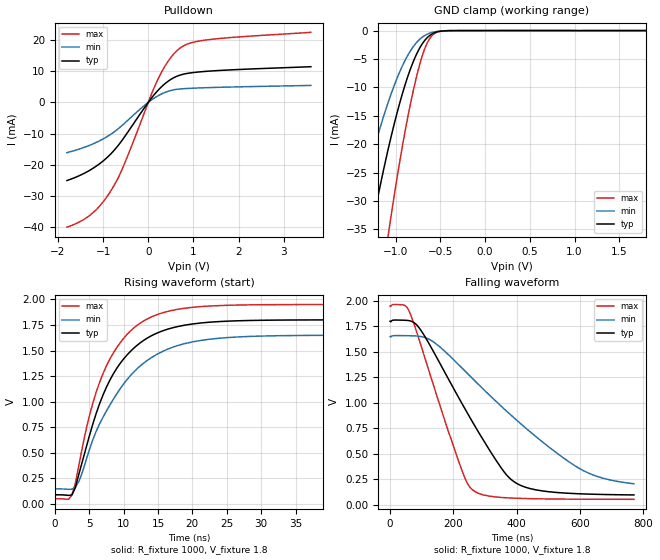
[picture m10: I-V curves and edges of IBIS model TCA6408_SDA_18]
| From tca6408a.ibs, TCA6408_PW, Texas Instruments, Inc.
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[Model]   TCA6408_SDA_18
Model_type  I/O_open_drain
Vinl=0.495
Vinh=1.365
Enable   Active-Low
Vref =   1.8
Rref =   1000
Cref =   50p
Vmeas =   0.9
| variable   typ   min   max
C_comp   2.96pF   1.98pF   3.47pF
| C_pulldown   1.93pF   0.86pF   2.70pF
| C_tri-state   2.96pF   1.98pF   3.47pF
[Temperature Range]   40   100   -40
| Ambient temperature   25   85   -40
[Voltage range]   1.8   1.65   1.95
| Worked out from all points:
|   slope of the pulldown table from 0 to 0.27 V, typ, clamps not added: 57.8 ohm
|   GND clamp passes 1 mA (typ) near -0.63 V on its own axis
|   rising waveform, R_fixture 1000, V_fixture 1.8: 20-80 % time 6.45ns typ, 7.78ns min, 5.79ns max; typ from 0.089 V to 1.8 V
|   falling waveform, R_fixture 1000, V_fixture 1.8: 20-80 % time 190ns typ, 311ns min, 119ns max; typ from 1.8 V to 0.094 V
[GND Clamp]
| TCA6408_SDA_18
|   Voltage   I(typ)   I(min)   I(max)
-1.8V     -85.23mA   -59.03mA   -129.6mA
-1.475V   -52.85mA   -35.21mA   -83.87mA
-1.275V   -35.29mA   -22.64mA   -58.08mA
-1.075V   -20.23mA   -12.2mA    -35.04mA
-965mV    -13.31mA   -7.618mA   -23.97mA
-860mV    -7.844mA   -4.209mA   -14.81mA
-760mV    -3.915mA   -1.979mA   -7.656mA
-675mV    -1.722mA   -861.6uA   -3.173mA
-630mV    -990.4uA   -511.7uA   -1.658mA
-585mV    -515uA     -286.9uA   -750uA
-455mV    -48.62uA   -37.39uA   -47.18uA
1.8V      212.6pA    1.031uA    -1.64uA
[Pulldown]
| TCA6408_SDA_18
|   Voltage   I(typ)   I(min)   I(max)
-1.8V     -25.03mA   -16.11mA   -39.97mA
-1.255V   -21.4mA    -13.49mA   -35.72mA
-1.045V   -19.29mA   -12.06mA   -32.67mA
-825mV    -16.44mA   -10.17mA   -28.24mA
-550mV    -11.55mA   -7.013mA   -20.47mA
60mV      1.174mA    652.4uA    2.253mA
215mV     3.846mA    2.097mA    7.413mA
445mV     6.827mA    3.573mA    13.29mA
680mV     8.622mA    4.255mA    17.11mA
920mV     9.403mA    4.495mA    18.95mA
1.315V    9.977mA    4.717mA    20.05mA
3.6V      11.43mA    5.425mA    22.44mA
[Ramp]
| TCA6408_SDA_18
| variable   typ   min   max
dV/dt_r   1.03/6.45E-09   0.90/7.78E-09   1.14/5.79E-09
dV/dt_f   1.03/1.91E-07   0.87/3.13E-07   1.15/1.20E-07
R_load = 1000
[Rising Waveform]
| TCA6408_SDA_18
R_fixture =   1000
C_fixture =   0
L_fixture =   0
V_fixture =   1.8
V_fixture_min = 1.65
V_fixture_max = 1.95
|   Time   V(typ)   V(min)   V(max)
0s        88.84mV    146.6mV    50.31mV
2.5ns     88.57mV    143.6mV    87.23mV
3.5ns     291mV      218.4mV    375.7mV
4.5ns     535.6mV    416.2mV    710.7mV
6ns       880.9mV    707.1mV    1.089V
8ns       1.209V     965.8mV    1.415V
10ns      1.417V     1.172V     1.618V
15ns      1.674V     1.468V     1.854V
22.5ns    1.777V     1.61V      1.935V
520ns     1.8V       1.65V      1.95V
[Falling Waveform]
| TCA6408_SDA_18
R_fixture =   1000
C_fixture =   0
L_fixture =   0
V_fixture =   1.8
V_fixture_min = 1.65
V_fixture_max = 1.95
|   Time   V(typ)   V(min)   V(max)
0s        1.8V       1.65V      1.95V
43.5ns    1.81V      1.659V     1.958V
61ns      1.806V     1.658V     1.894V
103.5ns   1.683V     1.646V     1.505V
220ns     1.031V     1.363V     394.9mV
262ns     802.1mV    1.232V     140.4mV
359.5ns   323mV      941.2mV    67.59mV
411.5ns   188.9mV    796.1mV    60.09mV
607.5ns   104.2mV    337.2mV    52.05mV
770ns     93.87mV    203.5mV    50.79mV
